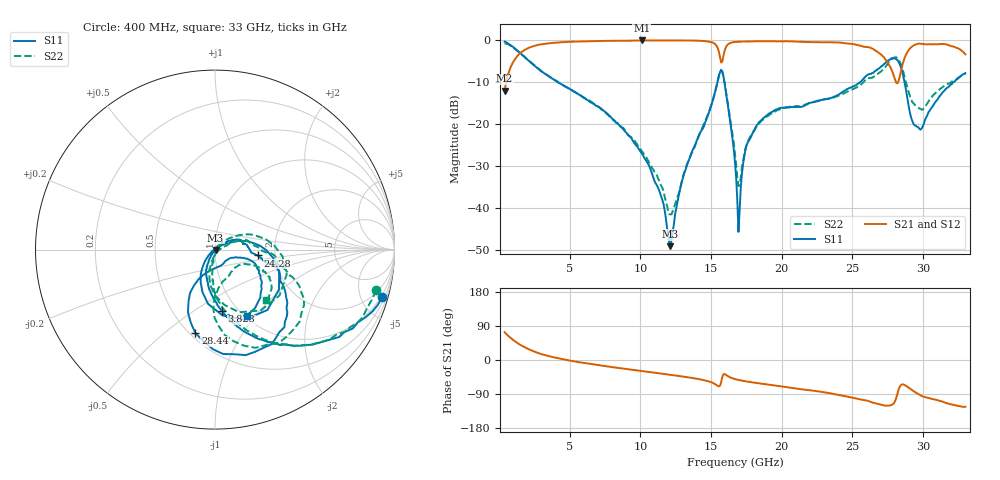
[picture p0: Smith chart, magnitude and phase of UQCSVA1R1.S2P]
!  Part Number  UQCSVA1R1  Mounting Orientation: Horizontal
!  Description: Ultra Low ESR Microwave capacitors
!  Application: Coupling, Bypass, Tuning, DC Block
!  Filters, Matching
# GHZ S DB R 50
! Freq  |S11|  S11 Ph  |S21|  S21 Ph  |S12|  S12 Ph  |S22|  S22 Ph
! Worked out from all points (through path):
!   401 points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, 400 MHz to 33 GHz, reference 50 ohm
!   highest |S21| = 0.00 dB at 10.1 GHz (marker M1); lowest = -12.0 dB at 400 MHz (marker M2)
!   group delay of S21, straight-line fit = 12.7 ps
!   lowest |S11| = -49.1 dB at 12.14 GHz (marker M3), VSWR 1.01, Z = 50.3 - j0.2 ohm
!   |S11| at or under -10 dB: 4.201 GHz to 15.46 GHz (11.26 GHz wide, 115 % of centre); 15.95 GHz to 25.54 GHz (9.584 GHz wide, 46.2 % of centre); 28.69 GHz to 32.14 GHz (3.446 GHz wide, 11.3 % of centre)
!   |S22| runs from -41.5 to -0.7 dB; largest |S21 - S12| = 0.013
!   S11 on the Smith chart (normalised r, x): 400 MHz: 0.81, -7.09; 3.823 GHz: 0.85, -0.66; 24.28 GHz: 1.62, -0.11; 28.44 GHz: 0.53, -0.64; 33 GHz: 1.03, -0.90
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0.4  -0.27 -15.9  -11.98 73.4  -12.22 75.5  -0.66 -14.2
1.46  -2.88 -48.2  -3.16 40.9  -3.15 41.4  -2.97 -48.6
3.823  -9.22 -83.4  -0.59 7.5  -0.58 7.4  -9.16 -80.5
5.861  -13.33 -99.2  -0.23 -6.8  -0.23 -6.7  -13.30 -92.2
10.099  -26.92 -122.3  0.00 -29.1  -0.01 -29.3  -26.43 -96.5
11.321  -35.67 -115.0  -0.01 -35.0  -0.01 -35.1  -33.36 -84.3
12.136  -49.11 -34.7  -0.01 -39.2  -0.01 -39.2  -41.53 -27.3
13.114  -31.64 34.2  -0.01 -44.2  -0.02 -44.3  -31.49 42.0
15.152  -14.10 12.7  -0.55 -60.8  -0.54 -60.7  -13.96 25.1
15.641  -7.53 -32.0  -4.00 -67.8  -3.96 -67.1  -7.48 -19.0
16.048  -12.09 -106.2  -1.66 -38.9  -1.64 -39.2  -11.90 -90.1
16.7  -29.12 -141.0  -0.37 -50.4  -0.35 -50.7  -27.04 -101.3
17.026  -40.71 72.9  -0.29 -53.1  -0.27 -53.4  -34.48 -20.4
17.434  -26.21 39.7  -0.23 -56.1  -0.23 -56.5  -25.78 19.9
18.33  -19.85 29.9  -0.20 -61.2  -0.26 -61.5  -20.04 23.3
22.161  -14.81 5.7  -0.40 -80.6  -0.37 -80.5  -14.72 16.5
24.28  -12.36 -7.7  -0.56 -94.1  -0.56 -94.0  -12.84 4.5
27.621  -4.68 -52.2  -5.96 -120.2  -5.94 -119.8  -4.98 -28.7
28.436  -6.42 -103.3  -7.40 -66.3  -7.37 -66.8  -5.67 -78.6
29.17  -18.54 -102.4  -1.60 -78.0  -1.62 -77.8  -14.07 -80.2
29.74  -21.06 -54.3  -0.75 -91.5  -0.77 -91.4  -16.25 -55.6
33  -7.80 -64.3  -3.31 -123.2  -3.31 -122.9  -7.97 -44.9
